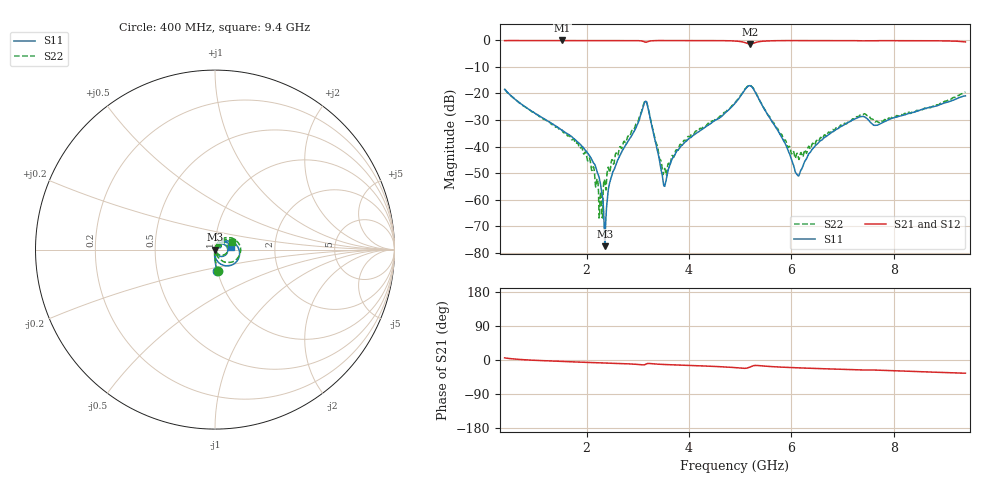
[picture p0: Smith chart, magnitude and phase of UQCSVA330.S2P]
!  Part Number  UQCSVA330  Mounting Orientation: Horizontal
!  Description: Ultra Low ESR Microwave capacitors
!  Application: Coupling, Bypass, Tuning, DC Block
!  Filters, Matching
# GHZ S DB R 50
! Freq  |S11|  S11 Ph  |S21|  S21 Ph  |S12|  S12 Ph  |S22|  S22 Ph
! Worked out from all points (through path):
!   801 points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, 400 MHz to 9.4 GHz, reference 50 ohm
!   highest |S21| = -0.01 dB at 1.525 GHz (marker M1); lowest = -1.3 dB at 5.193 GHz (marker M2)
!   group delay of S21, straight-line fit = 10.7 ps
!   lowest |S11| = -77.5 dB at 2.358 GHz (marker M3), VSWR 1.00, Z = 50 + j0.00916 ohm
!   |S11| at or under -10 dB: start of sweep to end of sweep
!   |S22| runs from -66.9 to -16.9 dB; largest |S21 - S12| = 0.0029
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0.4  -18.42 -84.7  -0.08 5.6  -0.06 5.6  -18.33 -83.2
1.525  -33.91 -96.3  -0.01 -3.9  -0.01 -4.0  -33.96 -93.5
1.908  -39.82 -99.2  -0.01 -5.8  0.00 -5.8  -40.36 -94.7
2.11  -45.27 -101.7  -0.01 -6.8  0.00 -6.8  -48.98 -82.3
2.279  -54.86 -105.6  -0.02 -7.5  -0.01 -7.5  -56.98 -15.0
2.358  -77.55 136.3  -0.02 -7.9  -0.01 -7.9  -53.13 37.1
2.526  -49.05 73.7  -0.02 -8.7  -0.01 -8.7  -46.64 65.5
3.134  -23.41 13.9  -0.55 -12.6  -0.54 -12.6  -23.05 23.3
3.201  -25.41 -45.9  -0.44 -9.1  -0.43 -9.2  -25.23 -33.8
3.404  -43.07 -74.8  -0.05 -11.1  -0.05 -11.1  -42.04 -60.0
3.528  -54.96 4.3  -0.04 -11.9  -0.03 -12.0  -48.25 7.9
3.674  -44.62 58.9  -0.03 -12.7  -0.03 -12.8  -43.32 60.5
3.865  -39.51 64.8  -0.03 -13.7  -0.02 -13.7  -39.28 75.1
4.9  -23.72 44.0  -0.22 -20.1  -0.22 -20.2  -23.49 58.2
5.193  -17.06 -20.7  -1.33 -18.4  -1.33 -18.4  -16.93 -5.4
5.834  -37.21 -94.0  -0.07 -19.0  -0.07 -19.1  -36.61 -69.7
6.115  -50.59 -33.4  -0.05 -20.6  -0.05 -20.7  -42.51 -15.3
6.408  -41.05 44.1  -0.05 -22.0  -0.05 -22.1  -38.96 39.1
7.296  -29.14 40.4  -0.11 -26.2  -0.11 -26.3  -28.75 44.3
7.645  -32.01 32.9  -0.13 -26.6  -0.14 -26.7  -30.69 30.5
7.904  -29.85 47.4  -0.07 -27.8  -0.08 -27.9  -29.25 43.4
9.4  -20.92 9.0  -0.56 -34.8  -0.57 -34.9  -19.47 24.0
